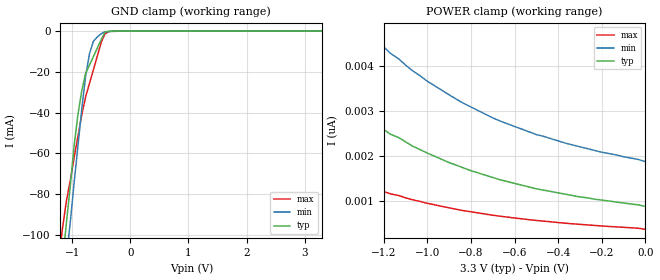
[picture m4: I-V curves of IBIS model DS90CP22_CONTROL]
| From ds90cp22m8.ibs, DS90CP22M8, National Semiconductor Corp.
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[Model]   DS90CP22_CONTROL
Model_type Input
Vinh=2.0
Vinl=0.8
C_comp   2.459pF   2.459pF   2.459pF
[Temperature Range] 25   85   -40
[Voltage Range]   3.3   3.0   3.6
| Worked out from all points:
|   GND clamp passes 1 mA (typ) near -0.44 V on its own axis
[GND Clamp]
-3.3V     -803mA     -823mA     -782mA
-1.17V    -114mA     -132mA     -97.7mA
-1.1V     -94.8mA    -112mA     -83.7mA
-1.03V    -75.7mA    -93.4mA    -73.1mA
-967mV    -56.7mA    -75mA      -62.4mA
-900mV    -41.1mA    -56.5mA    -51.8mA
-833mV    -29.2mA    -38.1mA    -41.1mA
-767mV    -20.7mA    -22.1mA    -32.2mA
-700mV    -16.6mA    -11mA      -25.6mA
-633mV    -12.5mA    -5.01mA    -18.9mA
-433mV    -470uA     -263uA     -1.31mA
3.3V      923pA      1.92nA     295pA
[POWER Clamp]
-3.3V     38.3nA     45.4nA     26.1nA
-2.17V    9.04nA     12.9nA     4.91nA
-2.13V    8.68nA     12.5nA     4.68nA
-2.07V    7.94nA     11.6nA     4.23nA
-1.87V    6.06nA     9.14nA     3.12nA
-1.7V     4.86nA     7.56nA     2.44nA
-1.47V    3.61nA     5.85nA     1.75nA
-1.27V    2.82nA     4.74nA     1.34nA
-1V       2.07nA     3.66nA     958pA
-700mV    1.53nA     2.85nA     695pA
-500mV    1.28nA     2.48nA     579pA
0V        889pA      1.88nA     383pA
